[IBIS Ver]   3.2
[File Name]   ixp46x_ibis.ibs
[File Rev]   0.00
[Date]   01/31/2006
[Source]   From silicon level SPICE model at Intel Corporation.
[Notes]   The following information corresponds to the ____ chip.
[Disclaimer]   This information is for modeling purposes only and is not
   guaranteed.
[Copyright]   Copyright 2004, Intel Corporation, All Rights Reserved.
[Define Package Model] Azusa
[Manufacturer] Intel Corp.
[OEM] xyz
[Description] Icemax Results
[Number Of Pins] 369
[Pin Numbers]
C5 |1 C5 DDR1_CB7
D5 |2 D5 DDR1_CB4
Y8 |3 Y8 ETHB_RXDATA3
AD2 |4 AD2 ETHB_RXCLK
D2 |5 D2 PCI_REQ_N1
F4 |6 F4 PCI_AD31
F5 |7 F5 PCI_GNT_N3
C2 |8 C2 PCI_GNT_N0
G6 |9 G6 PCI_INTA_N
H6 |10 H6 PCI_REQ_N2
Y5 |11 Y5 ETHB_TXEN
AC2 |12 AC2 ETHB_CRS
Y4 |13 Y4 ETHC_COL
E2 |14 E2 PCI_AD28
H4 |15 H4 PCI_AD24
G4 |16 G4 PCI_AD25
J5 |17 J5 PCI_AD23
F2 |18 F2 PCI_CBE_N3
Y3 |19 Y3 ETHC_RXDATA1
AA2 |20 AA2 ETHC_RXDATA0
G3 |21 G3 PCI_AD22
J4 |22 J4 PCI_AD19
V4 |23 V4 ETHC_TXDATA1
Y2 |24 Y2 ETHC_TXDATA0
W4 |25 W4 ETHC_RXDATA2
G2 |26 G2 PCI_AD20
H2 |27 H2 PCI_AD17
W2 |28 W2 ETHC_TXDATA3
J2 |29 J2 PCI_FRAME_N
V3 |30 V3 HSS_RXCLK1
J3 |31 J3 PCI_AD16
K4 |32 K4 PCI_STOP_N
U2 |33 U2 HSS_TXDATA1
V2 |34 V2 HSS_RXDATA1
L5 |35 L5 PCI_IRDY_N
L4 |36 L4 PCI_PAR
T3 |37 T3 HSS_RXFRAME0
K3 |38 K3 PCI_CBE_N2
K2 |39 K2 PCI_DEVSEL_N
M3 |40 M3 PCI_AD14
R2 |41 R2 PCI_AD5
L2 |42 L2 PCI_CBE_N1
L3 |43 L3 PCI_PERR_N
T4 |44 T4 HSS_RXDATA0
T2 |45 T2 HSS_TXCLK0
P3 |46 P3 PCI_AD2
R4 |47 R4 PCI_AD1
M2 |48 M2 PCI_AD12
P5 |49 P5 PCI_AD0
N2 |50 N2 PCI_AD4
N5 |51 N5 PCI_AD9
R3 |52 R3 PCI_AD3
P2 |53 P2 PCI_TRDY_N
H1 |54 H1 VCCP
G7 |55 G7 RCOMP_REF
F7 |56 F7 DDR1_CK2
H7 |57 H7 PCI_SERR_N
W7 |58 W7 ETHB_TXDATA0
U6 |59 U6 ETHC_RXDV
Y6 |60 Y6 ETHB_TXDATA1
W6 |61 W6 ETHB_COL
T6 |62 T6 ETHC_TXEN
J6 |63 J6 PCI_AD27
K6 |64 K6 PCI_IDSEL
H5 |65 H5 PCI_AD29
M4 |66 M4 PCI_AD13
N4 |67 N4 PCI_AD10
P4 |68 P4 PCI_AD8
E4 |69 E4 PCI_GNT_N2
C4 |70 C4 DDR1_CB5
M5 |71 M5 PCI_AD15
V5 |72 V5 ETHC_RXDATA3
G5 |73 G5 PCI_REQ_N3
T5 |74 T5 HSS_RXCLK0
U4 |75 U4 HSS_TXCLK1
D3 |76 D3 PCI_GNT_N1
R5 |77 R5 HSS_TXFRAME0
W5 |78 W5 ETHC_CRS
AA4 |79 AA4 ETHB_TXDATA3
E3 |80 E3 PCI_REQ_N0
AB3 |81 AB3 ETHB_TXDATA2
C1 |82 C1 PCI_AD30
AB2 |83 AB2 ETH_MDIO
AC1 |84 AC1 ETH_MDC
AD1 |85 AD1 ETHB_TXCLK
T1 |86 T1 HSS_TXDATA0
F1 |87 F1 PCI_AD21
R1 |88 R1 PCI_AD7
G1 |89 G1 PCI_AD18
E1 |90 E1 PCI_AD26
G8 |91 G8 DDR1_CK_N2
V6 |92 V6 VCC
AA1 |93 AA1 ETHC_TXCLK
V1 |94 V1 HSS_RXFRAME1
N1 |95 N1 PCI_AD6
L1 |96 L1 PCI_AD11
J1 |97 J1 PCI_CLKIN
Y1 |98 Y1 ETHC_TXDATA2
U1 |99 U1 HSS_TXFRAME1
AB1 |100 AB1 ETHC_RXCLK
M1 |101 M1 PCI_CBE_N0
A1 |102 A1 VSS
E7 |103 E7 VCCM
AE2 |104 AE2 UTP_OP_DATA6
AD3 |105 AD3 ETHB_RXDATA0
C3 |106 C3 DDR1_CB3
AF3 |107 AF3 UTP_OP_DATA0
B3 |108 B3 DDR1_CB2
A3 |109 A3 DDR1_CB0
AE3 |110 AE3 UTP_OP_DATA2
AC7 |111 AC7 UTP_OP_DATA3
B4 |112 B4 DDR1_CB1
AD4 |113 AD4 UTP_IP_DATA7
AE4 |114 AE4 UTP_OP_DATA1
AF4 |115 AF4 UTP_IP_DATA2
A4 |116 A4 DDR1_CK_N1
AC8 |117 AC8 UTP_IP_DATA5
AE5 |118 AE5 UTP_IP_DATA4
B5 |119 B5 DDR1_CK1
D7 |120 D7 DDR1_DM4
C6 |121 C6 DDR1_DQS4
A5 |122 A5 DDR1_DM3
D6 |123 D6 DDR1_CB6
AC6 |124 AC6 UTP_OP_DATA7
AD6 |125 AD6 UTP_IP_DATA6
B6 |126 B6 DDR1_DQS3
A6 |127 A6 DDR1_DQ30
AE6 |128 AE6 UTP_IP_DATA1
AF6 |129 AF6 UTP_IP_DATA0
D8 |130 D8 DDR1_DQ29
AA7 |131 AA7 ETHB_RXDV
C7 |132 C7 DDR1_DQ28
AB7 |133 AB7 ETHB_RXDATA2
B7 |134 B7 DDR1_DQ31
A7 |135 A7 DDR1_DQ26
AF7 |136 AF7 UTP_OP_CLK
AD8 |137 AD8 UTP_OP_SOC
C8 |138 C8 DDR1_DQ27
AA8 |139 AA8 ETHB_RXDATA1
AB8 |140 AB8 UTP_OP_DATA5
A8 |141 A8 DDR1_DQ25
AE8 |142 AE8 UTP_OP_ADDR4
AF8 |143 AF8 UTP_OP_ADDR2
B8 |144 B8 DDR1_DQ24
AD9 |145 AD9 UTP_OP_ADDR3
AA9 |146 AA9 UTP_OP_DATA4
AC9 |147 AC9 UTP_OP_FCO
AE9 |148 AE9 UTP_OP_ADDR1
C9 |149 C9 DDR1_DM2
B9 |150 B9 DDR1_DQ21
AF9 |151 AF9 UTP_OP_ADDR0
A9 |152 A9 DDR1_DQ22
D10 |153 D10 DDR1_DQS2
E11 |154 E11 DDR1_DQ20
AA10 |155 AA10 UTP_IP_DATA3
AD10 |156 AD10 UTP_IP_SOC
AB10 |157 AB10 UTP_OP_FCI
AC11 |158 AC11 UTP_IP_FCI
B10 |159 B10 DDR1_DQ23
AE10 |160 AE10 UTP_IP_FCO
A10 |161 A10 DDR1_DQ18
AF10 |162 AF10 UTP_IP_CLK
D11 |163 D11 DDR1_DQ19
AD11 |164 AD11 OSC_VCCP
AB11 |165 AB11 VCCPLL2
AF11 |166 AF11 OSC_IN
AE11 |167 AE11 OSC_VSSP
A11 |168 A11 DDR1_MA4
C11 |169 C11 DDR1_DQ16
B11 |170 B11 DDR1_DQ17
AB12 |171 AB12 VCCPLL3
AD12 |172 AD12 OSC_VSS
D12 |173 D12 DDR1_MA3
AC12 |174 AC12 VCCPLL1
B12 |175 B12 DDR1_MA5
E13 |176 E13 DDR1_MA2
D13 |177 D13 DDR1_MA6
C13 |178 C13 DDR1_MA1
B13 |179 B13 DDR1_MA7
AF13 |180 AF13 OSC_OUT
A13 |181 A13 DDR1_MA0
AD13 |182 AD13 OSC_VCC
AE13 |183 AE13 UTP_IP_ADDR3
AC13 |184 AC13 UTP_IP_ADDR4
AF14 |185 AF14 UTP_IP_ADDR2
A14 |186 A14 DDR1_MA8
AD14 |187 AD14 UTP_IP_ADDR0
AE14 |188 AE14 UTP_IP_ADDR1
D14 |189 D14 DDR1_MA10
B14 |190 B14 DDR1_MA9
AB14 |191 AB14 PLL_LOCK
AC14 |192 AC14 RESET_IN_N
AF15 |193 AF15 BYPASS_CLK
AF16 |194 AF16 PWRON_RESET_N
AE16 |195 AE16 SCANTESTMODE_N
A15 |196 A15 DDR1_BA1
AF17 |197 AF17 HIGHZ_N
E15 |198 E15 DDR1_MA12
B15 |199 B15 DDR1_MA11
AC15 |200 AC15 JTG_TMS
AD16 |201 AD16 JTG_TDI
C15 |202 C15 DDR1_BA0
AE17 |203 AE17 JTG_TDO
AF18 |204 AF18 JTG_TRST_N
D15 |205 D15 DDR1_MA13
AC16 |206 AC16 JTG_TCK
B16 |207 B16 DDR1_CS_N0
AD17 |208 AD17 TXDATA1
A17 |209 A17 DDR1_CS_N1
AE18 |210 AE18 RXDATA1
AF20 |211 AF20 CTS_N1
C16 |212 C16 DDR1_CKE0
D16 |213 D16 DDR1_CKE1
AE19 |214 AE19 RTS_N1
AD18 |215 AD18 TXDATA0
E17 |216 E17 DDR1_RCVENIN_N
B17 |217 B17 DDR1_RAS_N
E16 |218 E16 DDR1_WE_N
A18 |219 A18 DDR1_CAS_N
AC17 |220 AC17 CTS_N0
AB16 |221 AB16 RXDATA0
C17 |222 C17 DDR1_CK0
AE21 |223 AE21 GPIO15
AE20 |224 AE20 RTS_N0
D17 |225 D17 DDR1_CK_N0
AD20 |226 AD20 GPIO13
AC18 |227 AC18 GPIO14
B18 |228 B18 DDR1_VREF
AF22 |229 AF22 GPIO11
AB17 |230 AB17 GPIO12
C18 |231 C18 DDR1_RCVENOUT_N
A19 |232 A19 DDR1_DM1
AC19 |233 AC19 GPIO9
AF23 |234 AF23 GPIO10
B19 |235 B19 DDR1_DQS1
AA17 |236 AA17 GPIO7
D18 |237 D18 DDR1_DQ12
AB18 |238 AB18 GPIO8
A20 |239 A20 DDR1_DQ13
AD21 |240 AD21 GPIO5
B20 |241 B20 DDR1_DQ14
AE22 |242 AE22 GPIO6
C19 |243 C19 DDR1_DQ15
AF24 |244 AF24 GPIO3
AC20 |245 AC20 GPIO4
A21 |246 A21 DDR1_DQ11
AA18 |247 AA18 GPIO1
C20 |248 C20 DDR1_DQ10
AE23 |249 AE23 GPIO2
D19 |250 D19 DDR1_DQ9
AE24 |251 AE24 SSP_SCLK
D20 |252 D20 DDR1_DQ8
AD22 |253 AD22 GPIO0
A22 |254 A22 DDR1_DM0
AC21 |255 AC21 SSP_TXD
B21 |256 B21 DDR1_DQS0
AD23 |257 AD23 SSP_SFRM
AE25 |258 AE25 SSP_EXTCLK
C21 |259 C21 DDR1_DQ4
AA19 |260 AA19 SSP_RXD
B22 |261 B22 DDR1_DQ5
AD24 |262 AD24 I2C_SCL
A23 |263 A23 DDR1_DQ6
AB20 |264 AB20 I2C_SDA
B23 |265 B23 DDR1_DQ7
AC22 |266 AC22 EX_ADDR15
C22 |267 C22 DDR1_DQ3
AD25 |268 AD25 EX_ADDR16
Y19 |269 Y19 EX_ADDR13
C23 |270 C23 DDR1_DQ2
D22 |271 D22 DDR1_DQ1
AA20 |272 AA20 EX_ADDR14
D23 |273 D23 DDR1_DQ0
G20 |274 G20 DDR1_RCOMP
Y20 |275 Y20 EX_ADDR11
E23 |276 E23 USB_HPWR
AA22 |277 AA22 EX_ADDR0
B25 |278 B25 USB_HPEN
AC24 |279 AC24 EX_ADDR9
W20 |280 W20 EX_ADDR12
G22 |281 G22 USB_HPOS
Y22 |282 Y22 EX_ADDR7
D24 |283 D24 EX_CS_N1
AB24 |284 AB24 EX_PARITY0
Y21 |285 Y21 EX_ADDR10
H20 |286 H20 USB_DNEG
E24 |287 E24 EX_CS_N3
AC25 |288 AC25 EX_DATA0
G21 |289 G21 USB_DPOS
AB23 |290 AB23 EX_ADDR1
C26 |291 C26 EX_CS_N5
Y23 |292 Y23 EX_DATA1
H21 |293 H21 USB_HNEG
AD26 |294 AD26 EX_ADDR8
H22 |295 H22 EX_CS_N7
W22 |296 W22 EX_DATA2
F24 |297 F24 EX_GNT_REQ_N
F23 |298 F23 EX_CS_N0
AB26 |299 AB26 EX_DATA3
W21 |300 W21 EX_ADDR6
K21 |301 K21 EX_GNT_N2
Y24 |302 Y24 EX_DATA4
C25 |303 C25 EX_CS_N2
AA23 |304 AA23 EX_PARITY3
G24 |305 G24 EX_REQ_GNT_N
Y25 |306 Y25 EX_DATA5
E26 |307 E26 EX_REQ_N2
V23 |308 V23 EX_DATA6
D25 |309 D25 EX_CS_N4
AB25 |310 AB25 EX_DATA24
J23 |311 J23 EX_ADDR24
Y26 |312 Y26 EX_DATA7
J21 |313 J21 EX_CS_N6
G25 |314 G25 EX_ADDR22
V24 |315 V24 EX_DATA8
V21 |316 V21 EX_DATA25
J24 |317 J24 EX_ADDR20
W26 |318 W26 EX_DATA9
G23 |319 G23 EX_SLAVE_CS_N
G26 |320 G26 EX_ADDR18
V25 |321 V25 EX_DATA10
AA24 |322 AA24 EX_DATA26
J25 |323 J25 EX_ADDR5
T23 |324 T23 EX_DATA11
E25 |325 E25 EX_GNT_N1
L23 |326 L23 EX_ALE
U25 |327 U25 EX_DATA12
AA25 |328 AA25 EX_DATA27
M22 |329 M22 EX_WR_N
T25 |330 T25 EX_DATA13
L24 |331 L24 EX_BE_N0
T26 |332 T26 EX_DATA14
R25 |333 R25 EX_DATA15
L25 |334 L25 EX_BE_N2
H23 |335 H23 EX_GNT_N3
N22 |336 N22 EX_ADDR3
P23 |337 P23 EX_PARITY1
M25 |338 M25 EX_IOWAIT_N
P25 |339 P25 EX_BURST
U21 |340 U21 EX_DATA28
N24 |341 N24 EX_RDY_N1
N26 |342 N26 EX_RDY_N3
F25 |343 F25 EX_REQ_N1
W24 |344 W24 EX_DATA29
K22 |345 K22 EX_REQ_N3
U22 |346 U22 EX_DATA30
H24 |347 H24 EX_ADDR23
W25 |348 W25 EX_DATA31
H25 |349 H25 EX_ADDR21
U23 |350 U23 EX_DATA16
K23 |351 K23 EX_ADDR19
T22 |352 T22 EX_DATA17
H26 |353 H26 EX_ADDR17
U24 |354 U24 EX_DATA18
K24 |355 K24 EX_ADDR4
V26 |356 V26 EX_DATA19
K25 |357 K25 EX_RD_N
U26 |358 U26 EX_DATA20
K26 |359 K26 EX_CLK
R23 |360 R23 EX_DATA21
M23 |361 M23 EX_BE_N1
R24 |362 R24 EX_DATA22
L26 |363 L26 EX_BE_N3
P22 |364 P22 EX_DATA23
P24 |365 P24 EX_PARITY2
N23 |366 N23 EX_ADDR2
M26 |367 M26 EX_RDY_N0
P26 |368 P26 EX_WAIT_N
N25 |369 N25 EX_RDY_N2
[Model Data]
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[End Model Data]
[End Package Model]
[Component]   AZUSA
[Manufacturer]  Intel Corporation
[Package]
|   typ   min   max
R_pkg   130.000mOhm   80.000mOhm   260.000mOhm
L_pkg   5.00nH   4.00nH   7.00nH
C_pkg   1.10pF   800.00fF   2.00pF
[PIN] signal_name model_name R_pin L_pin C_pin
U1   HSS_TXFRAME1   gpio6x
V1   HSS_RXFRAME1   gpio6x
U2   HSS_TXDATA1   gpio6x
V2   HSS_RXDATA1   gpio6x
R5   HSS_TXFRAME0   gpio6x
T3   HSS_RXFRAME0   gpio6x
T1   HSS_TXDATA0   gpio6x
T4   HSS_RXDATA0   gpio6x
AC6   UTP_OP_DATA[7]  utp_mii_smii
AD4   UTP_IP_DATA[7]  utp_mii_smii
AE2   UTP_OP_DATA[6]  utp_mii_smii
AB8   UTP_OP_DATA[5]  utp_mii_smii
AA9   UTP_OP_DATA[4]  utp_mii_smii
AC7   UTP_OP_DATA[3]  utp_mii_smii
AE3   UTP_OP_DATA[2]  utp_mii_smii
AE4   UTP_OP_DATA[1]  utp_mii_smii
AF3   UTP_OP_DATA[0]  utp_mii_smii
AD6   UTP_IP_DATA[6]  utp_mii_smii
AC8   UTP_IP_DATA[5]  utp_mii_smii
AE5   UTP_IP_DATA[4]  utp_mii_smii
AA10   UTP_IP_DATA[3]  utp_mii_smii
AF4   UTP_IP_DATA[2]  utp_mii_smii
AE6   UTP_IP_DATA[1]  utp_mii_smii
AF6   UTP_IP_DATA[0]  utp_mii_smii
AC9   UTP_OP_FCO   utp_mii_smii
AD8   UTP_OP_SOC   utp_mii_smii
AB10   UTP_OP_FCI   utp_mii_smii
AF7   UTP_OP_CLK   utp_mii_smii
AE8   UTP_OP_ADDR[4]  utp_mii_smii
AD9   UTP_OP_ADDR[3]  utp_mii_smii
AF8   UTP_OP_ADDR[2]  utp_mii_smii
AE9   UTP_OP_ADDR[1]  utp_mii_smii
AF9   UTP_OP_ADDR[0]  utp_mii_smii
AD10   UTP_IP_SOC   utp_mii_smii
AC11   UTP_IP_FCI   utp_mii_smii
AE10   UTP_IP_FCO   utp_mii_smii
AF10   UTP_IP_CLK   utp_mii_smii
AC13   UTP_IP_ADDR[4]  utp_mii_smii
AE13   UTP_IP_ADDR[3]  utp_mii_smii
AF14   UTP_IP_ADDR[2]  utp_mii_smii
AE14   UTP_IP_ADDR[1]  utp_mii_smii
AD14   UTP_IP_ADDR[0]  utp_mii_smii
AC14   RESET_IN_N   gpio4x
AF15   BYPASS_CLK   gpio4x
AB14   PLL_LOCK   gpio4x
AE16   SCANTESTMODE_N  gpio4x
AF17   HIGHZ_N   gpio4x
AC15   JTG_TMS   gpio4x
AD16   JTG_TDI   gpio4x
AE17   JTG_TDO   gpio4x
AF18   JTG_TRST_N   gpio4x
AC16   JTG_TCK   gpio4x
AD17   TXDATA[1]   gpio4x
AE18   RXDATA[1]   gpio4x
AF20   CTS_N[1]   gpio4x
AE19   RTS_N[1]   gpio4x
AD18   TXDATA[0]   gpio4x
AB16   RXDATA[0]   gpio4x
AC17   CTS_N[0]   gpio4x
AE20   RTS_N[0]   gpio4x
AE21   GPIO[15]   gpio4x
AC18   GPIO[14]   gpio4x
AD20   GPIO[13]   gpio16x
AB17   GPIO[12]   gpio16x
AF22   GPIO[11]   gpio16x
AF23   GPIO[10]   gpio16x
AC19   GPIO[9]   gpio16x
AB18   GPIO[8]   gpio16x
AA17   GPIO[7]   gpio16x
AE22   GPIO[6]   gpio16x
AD21   GPIO[5]   gpio16x
AC20   GPIO[4]   gpio16x
AF24   GPIO[3]   gpio16x
AE23   GPIO[2]   gpio16x
AA18   GPIO[1]   gpio16x
AD22   GPIO[0]   gpio16x
AD23   SSP_SFRM   spi
AC21   SSP_TXD   spi
AA19   SSP_RXD   spi
AE24   SSP_SCLK   spi
AE25   SSP_EXTCLK   spi
AB20   I2C_SDA   gpio4x
AD24   I2C_SCL   gpio4x
P25   EX_BURST   exp_buf
P26   EX_WAIT_N   exp_buf
AA23   EX_PARITY[3]   exp_buf
P24   EX_PARITY[2]   exp_buf
P23   EX_PARITY[1]   exp_buf
AB24   EX_PARITY[0]   exp_buf
W25   EX_DATA[31]   exp_buf
U22   EX_DATA[30]   exp_buf
W24   EX_DATA[29]   exp_buf
U21   EX_DATA[28]   exp_buf
AA25   EX_DATA[27]   exp_buf
AA24   EX_DATA[26]   exp_buf
V21   EX_DATA[25]   exp_buf
AB25   EX_DATA[24]   exp_buf
P22   EX_DATA[23]   exp_buf
R24   EX_DATA[22]   exp_buf
R23   EX_DATA[21]   exp_buf
U26   EX_DATA[20]   exp_buf
V26   EX_DATA[19]   exp_buf
U24   EX_DATA[18]   exp_buf
T22   EX_DATA[17]   exp_buf
U23   EX_DATA[16]   exp_buf
R25   EX_DATA[15]   exp_buf
T26   EX_DATA[14]   exp_buf
T25   EX_DATA[13]   exp_buf
U25   EX_DATA[12]   exp_buf
T23   EX_DATA[11]   exp_buf
V25   EX_DATA[10]   exp_buf
W26   EX_DATA[9]   exp_buf
V24   EX_DATA[8]   exp_buf
Y26   EX_DATA[7]   exp_buf
V23   EX_DATA[6]   exp_buf
Y25   EX_DATA[5]   exp_buf
Y24   EX_DATA[4]   exp_buf
AB26   EX_DATA[3]   exp_buf
W22   EX_DATA[2]   exp_buf
Y23   EX_DATA[1]   exp_buf
AC25   EX_DATA[0]   exp_buf
N26   EX_RDY_N[3]   exp_buf
N25   EX_RDY_N[2]   exp_buf
N24   EX_RDY_N[1]   exp_buf
M26   EX_RDY_N[0]   exp_buf
M25   EX_IOWAIT_N   exp_buf
K25   EX_RD_N   exp_buf
M22   EX_WR_N   exp_buf
K26   EX_CLK   exp_buf
J23   EX_ADDR[24]   exp_buf
H24   EX_ADDR[23]   exp_buf
G25   EX_ADDR[22]   exp_buf
H25   EX_ADDR[21]   exp_buf
J24   EX_ADDR[20]   exp_buf
K23   EX_ADDR[19]   exp_buf
G26   EX_ADDR[18]   exp_buf
H26   EX_ADDR[17]   exp_buf
AD25   EX_ADDR[16]   exp_buf
AC22   EX_ADDR[15]   exp_buf
AA20   EX_ADDR[14]   exp_buf
Y19   EX_ADDR[13]   exp_buf
W20   EX_ADDR[12]   exp_buf
Y20   EX_ADDR[11]   exp_buf
Y21   EX_ADDR[10]   exp_buf
AC24   EX_ADDR[9]   exp_buf
AD26   EX_ADDR[8]   exp_buf
Y22   EX_ADDR[7]   exp_buf
W21   EX_ADDR[6]   exp_buf
J25   EX_ADDR[5]   exp_buf
K24   EX_ADDR[4]   exp_buf
N22   EX_ADDR[3]   exp_buf
N23   EX_ADDR[2]   exp_buf
AB23   EX_ADDR[1]   exp_buf
AA22   EX_ADDR[0]   exp_buf
L23   EX_ALE   exp_buf
K22   EX_REQ_N[3]   exp_buf
E26   EX_REQ_N[2]   exp_buf
F25   EX_REQ_N[1]   exp_buf
G24   EX_REQ_GNT_N   exp_buf
H23   EX_GNT_N[3]   exp_buf
K21   EX_GNT_N[2]   exp_buf
E25   EX_GNT_N[1]   exp_buf
F24   EX_GNT_REQ_N   exp_buf
G23   EX_SLAVE_CS_N   exp_buf
L26   EX_BE_N[3]   exp_buf
L25   EX_BE_N[2]   exp_buf
M23   EX_BE_N[1]   exp_buf
L24   EX_BE_N[0]   exp_buf
H22   EX_CS_N[7]   exp_buf
J21   EX_CS_N[6]   exp_buf
C26   EX_CS_N[5]   exp_buf
D25   EX_CS_N[4]   exp_buf
E24   EX_CS_N[3]   exp_buf
C25   EX_CS_N[2]   exp_buf
D24   EX_CS_N[1]   exp_buf
F23   EX_CS_N[0]   exp_buf
D23   DDR1_DQ[0]   ddr
D22   DDR1_DQ[1]   ddr
C23   DDR1_DQ[2]   ddr
C22   DDR1_DQ[3]   ddr
B21   DDR1_DQS[0]   ddr
C21   DDR1_DQ[4]   ddr
B22   DDR1_DQ[5]   ddr
A23   DDR1_DQ[6]   ddr
B23   DDR1_DQ[7]   ddr
A22   DDR1_DM[0]   ddr
C19   DDR1_DQ[15]   ddr
B20   DDR1_DQ[14]   ddr
A20   DDR1_DQ[13]   ddr
D18   DDR1_DQ[12]   ddr
B19   DDR1_DQS[1]   ddr
A21   DDR1_DQ[11]   ddr
C20   DDR1_DQ[10]   ddr
D19   DDR1_DQ[9]   ddr
D20   DDR1_DQ[8]   ddr
A19   DDR1_DM[1]   ddr
C18   DDR1_RCVENOUT_N ddr
B18   DDR1_VREF   ddr
E17   DDR1_RCVENIN_N  ddr
D17   DDR1_CK_N[0]   ddrmclk
C17   DDR1_CK[0]   ddrmclk
C11   DDR1_DQ[16]   ddr
B11   DDR1_DQ[17]   ddr
A10   DDR1_DQ[18]   ddr
D11   DDR1_DQ[19]   ddr
D10   DDR1_DQS[2]   ddr
E11   DDR1_DQ[20]   ddr
B9   DDR1_DQ[21]   ddr
A9   DDR1_DQ[22]   ddr
B10   DDR1_DQ[23]   ddr
C9   DDR1_DM[2]   ddr
B7   DDR1_DQ[31]   ddr
A6   DDR1_DQ[30]   ddr
D8   DDR1_DQ[29]   ddr
C7   DDR1_DQ[28]   ddr
B6   DDR1_DQS[3]   ddr
C8   DDR1_DQ[27]   ddr
A7   DDR1_DQ[26]   ddr
A8   DDR1_DQ[25]   ddr
B8   DDR1_DQ[24]   ddr
A5   DDR1_DM[3]   ddr
E16   DDR1_WE_N   ddr
A18   DDR1_CAS_N   ddr
D16   DDR1_CKE[1]   ddr
C16   DDR1_CKE[0]   ddr
B17   DDR1_RAS_N   ddr
A17   DDR1_CS_N[1]   ddr
B16   DDR1_CS_N[0]   ddr
D15   DDR1_MA[13]   ddr
E15   DDR1_MA[12]   ddr
C15   DDR1_BA[0]   ddr
A15   DDR1_BA[1]   ddr
B15   DDR1_MA[11]   ddr
B14   DDR1_MA[9]   ddr
D14   DDR1_MA[10]   ddr
A14   DDR1_MA[8]   ddr
A13   DDR1_MA[0]   ddr
B13   DDR1_MA[7]   ddr
C13   DDR1_MA[1]   ddr
D13   DDR1_MA[6]   ddr
E13   DDR1_MA[2]   ddr
B12   DDR1_MA[5]   ddr
D12   DDR1_MA[3]   ddr
A11   DDR1_MA[4]   ddr
C5   DDR1_CB[7]   ddr
A3   DDR1_CB[0]   ddr
D6   DDR1_CB[6]   ddr
B4   DDR1_CB[1]   ddr
C6   DDR1_DQS[4]   ddr
C4   DDR1_CB[5]   ddr
B3   DDR1_CB[2]   ddr
D5   DDR1_CB[4]   ddr
C3   DDR1_CB[3]   ddr
D7   DDR1_DM[4]   ddr
A4   DDR1_CK_N[1]   ddrmclk
B5   DDR1_CK[1]   ddrmclk
G8   DDR1_CK_N[2]   ddrmclk
F7   DDR1_CK[2]   ddrmclk
H7   PCI_SERR_N   pciod
G6   PCI_INTA_N   pciod
F5   PCI_GNT_N[3]   pci
E4   PCI_GNT_N[2]   pci
D3   PCI_GNT_N[1]   pci
C2   PCI_GNT_N[0]   pci
G5   PCI_REQ_N[3]   pci
H6   PCI_REQ_N[2]   pci
D2   PCI_REQ_N[1]   pci
E3   PCI_REQ_N[0]   pci
F4   PCI_AD[31]   pci
C1   PCI_AD[30]   pci
H5   PCI_AD[29]   pci
E2   PCI_AD[28]   pci
J6   PCI_AD[27]   pci
E1   PCI_AD[26]   pci
G4   PCI_AD[25]   pci
F2   PCI_CBE_N[3]   pci
H4   PCI_AD[24]   pci
K6   PCI_IDSEL   pci
J5   PCI_AD[23]   pci
G3   PCI_AD[22]   pci
F1   PCI_AD[21]   pci
G2   PCI_AD[20]   pci
J4   PCI_AD[19]   pci
G1   PCI_AD[18]   pci
H2   PCI_AD[17]   pci
J3   PCI_AD[16]   pci
J2   PCI_FRAME_N   pci
J1   PCI_CLKIN   pci
K4   PCI_STOP_N   pci
K3   PCI_CBE_N[2]   pci
L5   PCI_IRDY_N   pci
K2   PCI_DEVSEL_N   pci
L4   PCI_PAR   pci
L3   PCI_PERR_N   pci
M5   PCI_AD[15]   pci
L2   PCI_CBE_N[1]   pci
L1   PCI_AD[11]   pci
M4   PCI_AD[13]   pci
M3   PCI_AD[14]   pci
M2   PCI_AD[12]   pci
M1   PCI_CBE_N[0]   pci
N5   PCI_AD[9]   pci
N4   PCI_AD[10]   pci
N2   PCI_AD[4]   pci
N1   PCI_AD[6]   pci
P2   PCI_TRDY_N   pci
P3   PCI_AD[2]   pci
P4   PCI_AD[8]   pci
P5   PCI_AD[0]   pci
R1   PCI_AD[7]   pci
R2   PCI_AD[5]   pci
R3   PCI_AD[3]   pci
R4   PCI_AD[1]   pci
Y5   ETHB_TXEN   mii_smii
AA4   ETHB_TXDATA[3]  mii_smii
AB3   ETHB_TXDATA[2]  mii_smii
Y6   ETHB_TXDATA[1]  mii_smii
W7   ETHB_TXDATA[0]  mii_smii
AD1   ETHB_TXCLK   mii_smii
AA7   ETHB_RXDV   mii_smii
Y8   ETHB_RXDATA[3]  mii_smii
AB7   ETHB_RXDATA[2]  mii_smii
AA8   ETHB_RXDATA[1]  mii_smii
AD3   ETHB_RXDATA[0]  mii_smii
AD2   ETHB_RXCLK   mii_smii
AC2   ETHB_CRS   mii_smii
W6   ETHB_COL   mii_smii
AB2   ETH_MDIO   gpio6x
AC1   ETH_MDC   gpio6x
T6   ETHC_TXEN   mii_smii
W2   ETHC_TXDATA[3]  mii_smii
Y1   ETHC_TXDATA[2]  mii_smii
V4   ETHC_TXDATA[1]  mii_smii
Y2   ETHC_TXDATA[0]  mii_smii
AA1   ETHC_TXCLK   mii_smii
U6   ETHC_RXDV   mii_smii
V5   ETHC_RXDATA[3]  mii_smii
W4   ETHC_RXDATA[2]  mii_smii
Y3   ETHC_RXDATA[1]  mii_smii
AA2   ETHC_RXDATA[0]  mii_smii
AB1   ETHC_RXCLK   mii_smii
W5   ETHC_CRS   mii_smii
Y4   ETHC_COL   mii_smii
U4   HSS_TXCLK1   gpio6x
V3   HSS_RXCLK1   gpio6x
T2   HSS_TXCLK0   gpio6x
T5   HSS_RXCLK0   gpio6x
B25   USB_HPEN   exp_buf
E23   USB_HPWR   exp_buf
|**********************DIFF PIN*********************************************
[Diff_pin]   inv_pin   vdiff   tdelay_typ   tdelay_min   tdelay_max
   C17   D17   .400V   0ns   NA   NA
   B5   A4   .400V   0ns   NA   NA
   F7   G8   .400V   0ns   NA   NA
|***********************MODEL SELECTOR**************************************
[Model Selector] utp_mii_smii
gpio8x   Drive Strength for Utopia
gpio6x   Drive Strength for MII/RMII
smii   Drive strength for SMII mode
|***********************MODEL SELECTOR**************************************
[Model Selector] mii_smii
gpio6x   Drive Strength for MII/RMII
smii   Drive strength for SMII mode
|***********************MODEL SELECTOR**************************************
[Model Selector] exp_buf
gpio8x   Low-Strength IO Driver
gpio14x   Medium-Strength IO Driver
gpio20x   High-Strength IO Driver
| Models and submodels in the file (12): gpio4x (I/O), gpio6x (I/O), gpio16x (I/O), smii (I/O), spi (I/O), gpio8x (I/O), gpio14x (I/O), gpio20x (I/O), ddr (I/O), ddrmclk (Output), pciod (I/O_open_drain), pci (I/O)
